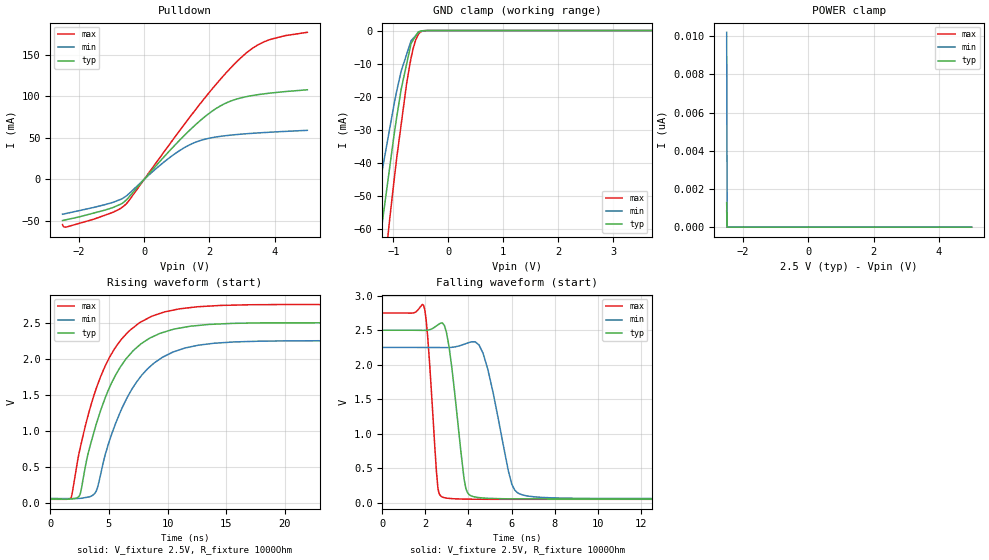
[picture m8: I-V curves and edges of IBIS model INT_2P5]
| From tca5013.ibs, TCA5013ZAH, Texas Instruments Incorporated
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[Model]   INT_2P5
Model_type   Open_drain
Polarity   Non-Inverting
Vmeas = 1.25
Vref = 2.5
Cref = 15pF
Rref = 1000
|   typ   min   max
C_comp   2.075p   1.623p   2.368p
|C_comp (Low state)   2.075p   1.623p   2.368p
|C_comp (High state)   2.147p   1.701p   2.380p
[Voltage Range]   2.5   2.25   2.75
[Temperature Range]   27   125   -40
[Pullup Reference]   2.5   2.25   2.75
[Pulldown Reference]   0   0   0
[Power Clamp Reference]   2.5   2.25   2.75
[GND Clamp Reference]   0   0   0
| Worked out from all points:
|   slope of the pulldown table from 0 to 0.375 V, typ, clamps not added: 22.2 ohm
|   GND clamp passes 1 mA (typ) near -0.57 V on its own axis
|   falling waveform, V_fixture 2.5V, R_fixture 1000Ohm: 20-80 % time 518ps typ, 843ps min, 332ps max; typ from 2.5 V to 0.051 V
|   rising waveform, V_fixture 2.5V, R_fixture 1000Ohm: 20-80 % time 3.5ns typ, 3.61ns min, 3.47ns max; typ from 0.051 V to 2.5 V
[Pulldown]
|   Voltage   I(typ)   I(min)   I(max)
-2.5V     -49.39mA   -41.82mA   -54.22mA
-2.395V   -48.51mA   -40.98mA   -57.36mA
-1.529V   -40.27mA   -33.53mA   -47.61mA
-550mV    -24.89mA   -19.96mA   -29.46mA
432.5mV   19.43mA    15.21mA    23.57mA
1.167V    50.32mA    36.66mA    62.78mA
1.722V    70.86mA    46.8mA     91.23mA
2.428V    90.28mA    52.25mA    124.4mA
3.058V    98.85mA    54.68mA    149.5mA
3.493V    101.9mA    55.89mA    161.9mA
4.325V    105.6mA    57.74mA    172.9mA
5V        107.7mA    59.02mA    176.8mA
[GND Clamp]
|   Voltage   I(typ)   I(min)   I(max)
-2.5V     -246.4mA   -197.1mA   -297.3mA
-1.383V   -82.65mA   -61.26mA   -107.2mA
-1.278V   -68.47mA   -50.23mA   -90.15mA
-1.202V   -58.34mA   -42.36mA   -78.44mA
-1.067V   -41.59mA   -29.83mA   -57.36mA
-940mV    -26.36mA   -18.42mA   -38.78mA
-857.5mV  -17.75mA   -12.3mA    -28.44mA
-760mV    -10.27mA   -7.318mA   -16.22mA
-677.5mV  -3.932mA   -3.098mA   -8.313mA
-542.5mV  -396.2uA   -612uA     -1.098mA
-362.5mV  -4.017uA   -15.05uA   -5.943uA
5V        0A         0A         0A
[POWER Clamp]
|   Voltage   I(typ)   I(min)   I(max)
-2.5V     1.287nA    10.2nA     852.5pA
-2.485V   0A         0A         0A
-2.478V   0A         0A         0A
5V        0A         0A         0A
[Ramp]
R_load = 1000
|   typ   min   max
dV/dt_r   1.4693/3.49868e-09   1.31529/3.6052e-09   1.62206/3.46562e-09
dV/dt_f   1.4693/5.1752e-10   1.31534/8.42941e-10   1.62206/3.31775e-10
[Falling Waveform]
V_fixture = 2.5V
V_fixture_min = 2.25V
V_fixture_max = 2.75V
R_fixture = 1000Ohm
C_fixture = 0F
|   Time   V(typ)   V(min)   V(max)
0s        2.5V       2.25V      2.75V
1.916ns   2.498V     2.25V      2.862V
2.58ns    2.578V     2.249V     212.7mV
2.991ns   2.445V     2.249V     63.96mV
3.796ns   338.6mV    2.297V     49.91mV
4.297ns   80.55mV    2.332V     48.03mV
4.897ns   61.66mV    1.934V     47.32mV
6.014ns   53.56mV    261.9mV    47.11mV
6.725ns   52.35mV    95.43mV    47.1mV
49.9ns    51.17mV    57.75mV    46.57mV
[Rising Waveform]
V_fixture = 2.5V
V_fixture_min = 2.25V
V_fixture_max = 2.75V
R_fixture = 1000Ohm
C_fixture = 0F
|   Time   V(typ)   V(min)   V(max)
0s        51.17mV    57.75mV    46.57mV
1.799ns   51.59mV    55.41mV    77.55mV
2.527ns   108.9mV    59.69mV    740.7mV
3.807ns   1.027V     130mV      1.529V
5.144ns   1.631V     906.9mV    2.043V
6.52ns    2.007V     1.447V     2.348V
7.821ns   2.213V     1.773V     2.515V
9.735ns   2.369V     2.031V     2.647V
15.64ns   2.489V     2.23V      2.741V
49.9ns    2.5V       2.25V      2.75V
